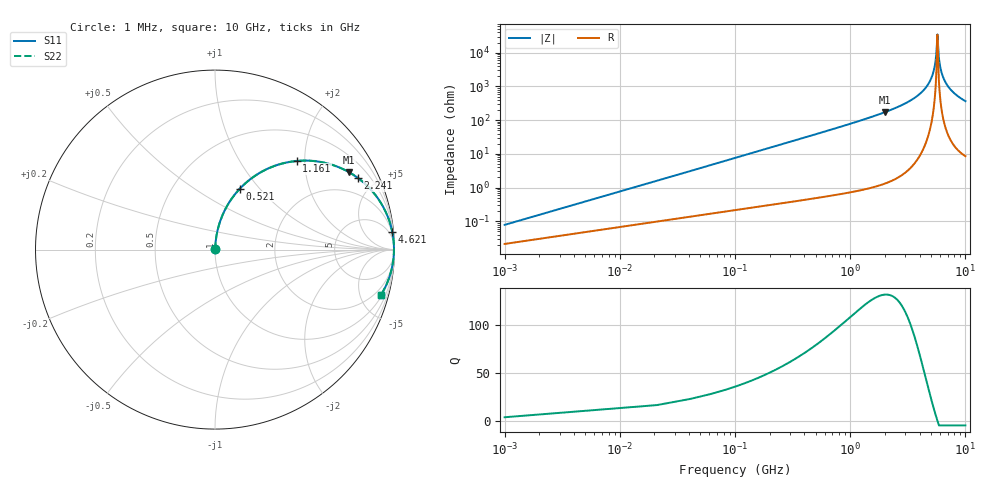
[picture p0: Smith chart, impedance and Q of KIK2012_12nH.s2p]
!version-2
!date-01.2022
!Series
# MHz S RI R 50
!Freq ReS11 ImS11 ReS21 ImS21 ReS12 ImS12 ReS22 ImS22
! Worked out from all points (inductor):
!   501 points, 1 MHz to 10 GHz, reference 50 ohm
!   read as one part in series: L = 12 nH near 41 MHz
!   highest Q = 131 at 2.001 GHz (marker M1), where L = 13.7 nH
!   self-resonance near 5.701 GHz
!   S11 on the Smith chart (normalised r, x): 1 MHz: 1.00, +0.00; 521 MHz: 1.01, +0.79; 1.161 GHz: 1.02, +1.83; 2.241 GHz: 1.03, +3.99; 4.621 GHz: 2, +20; 10 GHz: 1.17, -7.31
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1  0.000214 0.000754  0.9998 -0.000754  0.9998 -0.000754  0.000214 0.000754
61  0.00376 0.0457  0.9962 -0.0457  0.9962 -0.0457  0.00376 0.0457
121  0.0105 0.0901  0.9895 -0.0901  0.9895 -0.0901  0.0105 0.0901
281  0.0463 0.2018  0.9537 -0.2018  0.9537 -0.2018  0.0463 0.2018
521  0.1387 0.3395  0.8613 -0.3395  0.8613 -0.3395  0.1387 0.3395
1161  0.4551 0.4936  0.5449 -0.4936  0.5449 -0.4936  0.4551 0.4936
1681  0.657 0.4708  0.343 -0.4708  0.343 -0.4708  0.657 0.4708
2001  0.7457 0.4317  0.2543 -0.4317  0.2543 -0.4317  0.7457 0.4317
2241  0.7977 0.3979  0.2023 -0.3979  0.2023 -0.3979  0.7977 0.3979
3341  0.934 0.2434  0.066 -0.2434  0.066 -0.2434  0.934 0.2434
4621  0.9878 0.0979  0.0122 -0.0979  0.0122 -0.0979  0.9878 0.0979
5001  0.9936 0.0615  0.00637 -0.0615  0.00637 -0.0615  0.9936 0.0615
5461  0.9968 0.0209  0.00315 -0.0209  0.00315 -0.0209  0.9968 0.0209
5561  0.9971 0.0126  0.00291 -0.0126  0.00291 -0.0126  0.9971 0.0126
5681  0.9972 0.00271  0.00282 -0.00271  0.00282 -0.00271  0.9972 0.00271
5721  0.9972 -0.000526  0.00283 0.000526  0.00283 0.000526  0.9972 -0.000526
5861  0.997 -0.0117  0.00303 0.0117  0.00303 0.0117  0.997 -0.0117
6021  0.9964 -0.0241  0.00356 0.0241  0.00356 0.0241  0.9964 -0.0241
6281  0.995 -0.0436  0.00502 0.0436  0.00502 0.0436  0.995 -0.0436
6681  0.9914 -0.072  0.00858 0.072  0.00858 0.072  0.9914 -0.072
8341  0.9645 -0.1725  0.0355 0.1725  0.0355 0.1725  0.9645 -0.1725
10000  0.9253 -0.2514  0.0747 0.2514  0.0747 0.2514  0.9253 -0.2514
